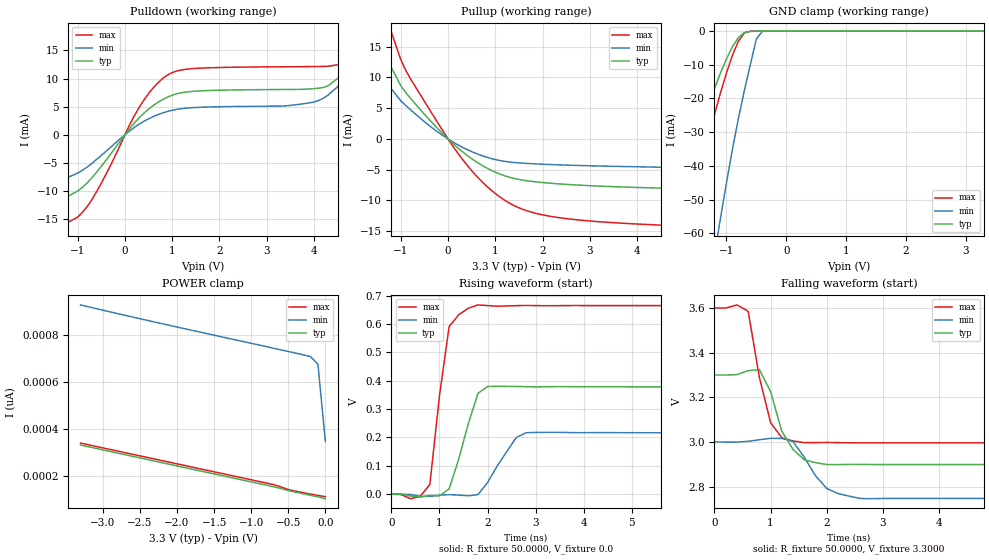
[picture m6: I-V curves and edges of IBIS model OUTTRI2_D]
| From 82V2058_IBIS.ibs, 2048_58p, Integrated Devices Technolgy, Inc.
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|   Model OUTTRI2_D
[Model]   OUTTRI2_D
Model_type   3-state
Polarity   Non-Inverting
Enable   Active-Low
Vmeas =   1.65V
C_comp   2.6600pF   2.5500pF   2.7500pF
[Temperature Range]   25.0000   85.0000   -40.0000
[Voltage Range]   3.3000V   3.0000V   3.6000V
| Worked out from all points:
|   slope of the pulldown table from 0 to 0.495 V, typ, clamps not added: 110 ohm
|   slope of the pullup table from 0 to 0.495 V, typ, clamps not added: 155 ohm
|   GND clamp passes 1 mA (typ) near -0.74 V on its own axis
|   rising waveform, R_fixture 50.0000, V_fixture 0.0: 20-80 % time 392ps typ, 483ps min, 289ps max; typ from 0 V to 0.378 V
|   falling waveform, R_fixture 50.0000, V_fixture 3.3000: 20-80 % time 363ps typ, 431ps min, 298ps max; typ from 3.3 V to 2.9 V
[Pulldown]
|Voltage   I(typ)   I(min)   I(max)
-3.3V     -12.6mA    -9.6mA     -16.6mA
-1.7V     -12.7mA    -9.1mA     -17.25mA
-1V       -10.05mA   -6.85mA    -14.7mA
-600mV    -6.689mA   -4.42mA    -10.16mA
400mV     3.821mA    2.375mA    6.161mA
1V        7.035mA    4.342mA    11.06mA
4V        8.205mA    5.815mA    12.14mA
4.5V      10.01mA    8.535mA    12.45mA
5.1V      17.96mA    14.06mA    20.72mA
5.3V      21.62mA    15.74mA    25.34mA
5.9V      34.85mA    19.63mA    42.76mA
6.6V      52.53mA    21.74mA    68.33mA
[Pullup]
|Voltage   I(typ)   I(min)   I(max)
-3.2V     55.48mA    28.48mA    77.76mA
-2V       26.64mA    17.85mA    39.13mA
-1.6V     18.26mA    12.6mA     27.24mA
-1.4V     14.57mA    10.09mA    21.83mA
-900mV    7.585mA    5.469mA    11.22mA
0V        -6.42pA    -41.9pA    -6.2pA
700mV     -4.208mA   -2.668mA   -6.814mA
1.1V      -5.713mA   -3.508mA   -9.453mA
1.5V      -6.585mA   -3.891mA   -11.2mA
2V        -7.084mA   -4.102mA   -12.34mA
2.8V      -7.516mA   -4.316mA   -13.2mA
6.6V      -8.6mA     -4.9mA     -15.1mA
[GND_clamp]
|Voltage   I(typ)   I(min)   I(max)
-3.3V     -132.9mA   -313.8mA   -170.5mA
-2V       -60.27mA   -158.7mA   -81.36mA
-1.9V     -54.57mA   -146.8mA   -74.16mA
-1.7V     -43.29mA   -123.2mA   -59.73mA
-1.2V     -17.04mA   -66.31mA   -24.76mA
-1.1V     -12.49mA   -55.54mA   -18.38mA
-900mV    -4.665mA   -35.06mA   -7.189mA
-800mV    -1.94mA    -25.89mA   -2.998mA
-700mV    -476.2uA   -17.58mA   -563.2uA
-500mV    -16.62uA   -2.324mA   -1.086uA
-400mV    -424.8nA   -91.35uA   -22.54nA
3.3V      102.4pA    717.1pA    94.7pA
[POWER_clamp]
|Voltage   I(typ)   I(min)   I(max)
-3.3V     331.5pA    929.7pA    339.8pA
-2.4V     269.7pA    863.7pA    278.5pA
-700mV    153.7pA    744.9pA    162.8pA
-500mV    137.1pA    730.9pA    141.3pA
-200mV    116.9pA    709.2pA    122.1pA
-100mV    110.2pA    677pA      116.6pA
0V        102.4pA    346.3pA    111.1pA
[Ramp]
| variable   typ   min   max
dV/dt_r   0.2269/0.3575n   0.1295/0.4806n   0.3988/0.2755n
dV/dt_f   0.2406/0.3125n   0.1518/0.4105n   0.3624/0.2421n
R_load =   50.0000
[Rising Waveform]
R_fixture=   50.0000
V_fixture=   0.0
V_fixture_min=  0.0
V_fixture_max=  0.0
|time   V(typ)   V(min)   V(max)
0s        0V         0V         0V
600ps     -10.38mV   -7.905mV   -7.895mV
800ps     -3.837mV   -7.972mV   34.55mV
1ns       -6.035mV   -3.304mV   347.2mV
1.2ns     18.19mV    -1.702mV   590.3mV
1.6ns     248.8mV    -5.845mV   655.2mV
1.8ns     355mV      -1.595mV   666.9mV
2ns       379.6mV    40.95mV    664.6mV
2.8ns     378.8mV    216.4mV    664.9mV
10ns      378.2mV    215.8mV    664.6mV
[Falling Waveform]
R_fixture=   50.0000
V_fixture=   3.3000
V_fixture_min=  3.0000
V_fixture_max=  3.6000
|time   V(typ)   V(min)   V(max)
0s        3.3V       3V         3.6V
600ps     3.319V     3.003V     3.585V
800ps     3.324V     3.01V      3.29V
1ns       3.225V     3.016V     3.086V
1.2ns     3.048V     3.016V     3.019V
1.4ns     2.966V     3.002V     3.005V
1.6ns     2.92V      2.932V     2.997V
2ns       2.899V     2.792V     2.998V
2.6ns     2.9V       2.747V     2.996V
10ns      2.899V     2.747V     2.996V
